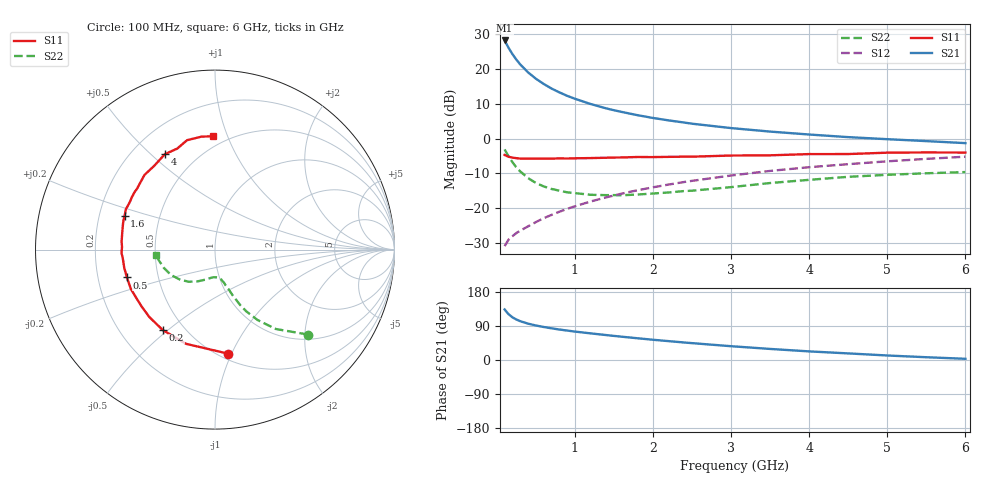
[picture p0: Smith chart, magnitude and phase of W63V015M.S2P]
! SIEMENS Small Signal Semiconductors
! BFR193W
! Si NPN RF Bipolar Junction Transistor in SOT323
! VCE = 3 V  IC = 15 mA
! Common Emitter S-Parameters:  September  1992
# GHz  S  MA  R  50
!  f  S11  S21  S12  S22
! GHz  MAG  ANG  MAG  ANG  MAG  ANG  MAG  ANG
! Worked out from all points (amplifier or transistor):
!   28 points, 100 MHz to 6 GHz, reference 50 ohm
!   highest |S21| = 28.2 dB at 100 MHz (marker M1)
!   |S21| within 3 dB of that: start of sweep to 175 MHz
!   unconditionally stable (mu >= 1): 841.6 MHz to 2.547 GHz
!   at 300 MHz: K = 0.69, MSG = 23.9 dB, |S12| = -26.4 dB
!   at 1.5 GHz: K = 1.04, MAG = 11.0 dB, |S12| = -16.3 dB
!   at 6 GHz: K = 0.91, MSG = 2.0 dB, |S12| = -5.2 dB
!   S11 on the Smith chart (normalised r, x): 100 MHz: 0.55, -0.97; 200 MHz: 0.38, -0.48; 500 MHz: 0.33, -0.14; 1.6 GHz: 0.31, +0.16; 4 GHz: 0.33, +0.55; 6 GHz: 0.42, +0.89
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0.1  0.5833 -83.1  25.79 133.4  0.0285 58.8  0.7017 -42.4
0.15  0.5492 -107.1  20.27 121.0  0.0353 54.2  0.5579 -52.5
0.2  0.5345 -122.9  16.44 112.7  0.0396 52.4  0.4591 -58.8
0.25  0.5245 -134.2  13.68 106.9  0.044 52.4  0.3862 -63.1
0.3  0.5172 -142.4  11.68 102.4  0.0476 53.5  0.3384 -65.6
0.4  0.5176 -154.6  8.974 95.9  0.0549 56.0  0.2712 -69.0
0.5  0.515 -162.5  7.278 91.1  0.0632 58.5  0.2313 -71.2
0.6  0.5157 -168.8  6.119 87.1  0.0719 60.4  0.206 -73.6
0.7  0.5156 -173.8  5.257 83.6  0.0802 62.0  0.1895 -75.0
0.8  0.5212 -178.1  4.634 80.5  0.0889 63.2  0.1788 -77.0
0.9  0.5182 178.4  4.131 77.7  0.0979 64.1  0.1694 -78.3
1  0.5222 175.1  3.749 75.0  0.1067 64.8  0.1649 -80.1
1.2  0.5259 169.2  3.151 70.3  0.1249 65.3  0.1561 -84.5
1.4  0.532 164.5  2.727 65.8  0.1433 65.5  0.1543 -88.4
1.6  0.537 159.8  2.421 61.5  0.1623 65.3  0.1538 -92.5
2.2  0.5477 147.6  1.831 49.8  0.219 63.2  0.1685 -103.9
3  0.5722 133.4  1.419 36.4  0.2954 58.3  0.2011 -118.5
3.5  0.5763 126.2  1.264 29.2  0.344 54.6  0.2304 -129.0
4  0.6004 117.7  1.147 22.7  0.389 50.2  0.256 -138.8
4.5  0.6009 110.5  1.052 17.4  0.43 46.1  0.2829 -150.0
5.5  0.6339 96.8  0.922 7.3  0.5124 37.5  0.3181 -168.9
6  0.6314 91.2  0.863 3.2  0.5507 32.8  0.3311 -175.1
